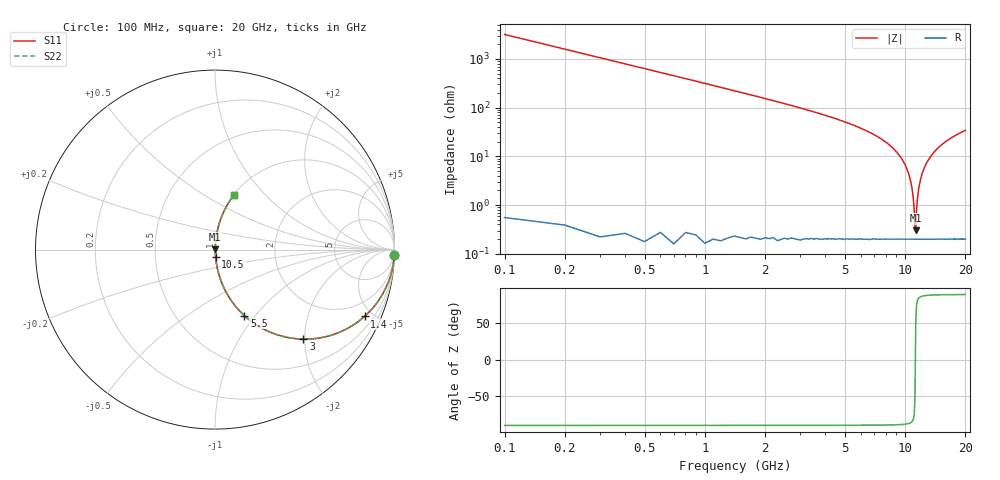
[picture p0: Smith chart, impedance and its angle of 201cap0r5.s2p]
! AVX Thin Film Operation		Date: May 2007
! Description: Accu-P® Series, Thin Film, SMD, RF Capacitor
! Part Number: 02013J0R5ABS
! 50 MHz  -  20.05 GHz
! Serial Measurements
# hz S db R 50
!	S11		S21		S12		S22
!	dB	Phase	dB	Phase	dB	Phase	dB	Phase
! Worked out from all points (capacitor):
!   200 points, 100 MHz to 20 GHz, reference 50 ohm
!   read as one part in series: C = 500 fF near 200 MHz
!   lowest |Z| = 305 mohm at 11.3 GHz (marker M1)
!   series resonance near 11.25 GHz, so ESL is about 400 pH
!   S11 on the Smith chart (normalised r, x): 100 MHz: 1, -64; 1.4 GHz: 1.00, -4.48; 3 GHz: 1.00, -1.97; 5.5 GHz: 1.00, -0.88; 10.5 GHz: 1.00, -0.08; 20 GHz: 1.00, +0.69
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1e8  -0.00 -1.8  -30.06 88.2  -30.06 88.2  -0.00 -1.8
3e8  -0.04 -5.4  -20.55 84.6  -20.55 84.6  -0.04 -5.4
5e8  -0.11 -8.9  -16.17 81.0  -16.17 81.0  -0.11 -8.9
1.4e9  -0.79 -24.1  -7.79 65.9  -7.79 65.9  -0.79 -24.1
3e9  -3.08 -45.4  -2.96 44.5  -2.96 44.5  -3.08 -45.4
3.5e9  -3.96 -50.5  -2.25 39.4  -2.25 39.4  -3.96 -50.5
5.5e9  -7.91 -66.0  -0.78 23.7  -0.78 23.7  -7.91 -66.0
6.8e9  -10.92 -73.1  -0.38 16.5  -0.38 16.5  -10.92 -73.1
8.8e9  -17.14 -81.2  -0.10 8.0  -0.10 8.0  -17.14 -81.2
1.01e10  -24.28 -84.6  -0.03 3.5  -0.03 3.5  -24.28 -84.6
1.05e10  -28.13 -84.8  -0.02 2.2  -0.02 2.2  -28.13 -84.8
1.09e10  -34.82 -82.7  -0.02 1.0  -0.02 1.0  -34.82 -82.7
1.11e10  -41.91 -75.2  -0.02 0.4  -0.02 0.4  -41.91 -75.2
1.12e10  -49.45 -53.5  -0.02 0.2  -0.02 0.2  -49.45 -53.5
1.13e10  -50.32 49.0  -0.02 -0.1  -0.02 -0.1  -50.32 49.0
1.14e10  -42.44 74.2  -0.02 -0.4  -0.02 -0.4  -42.44 74.2
1.15e10  -38.15 80.0  -0.02 -0.7  -0.02 -0.7  -38.15 80.0
1.18e10  -31.43 84.2  -0.02 -1.5  -0.02 -1.5  -31.43 84.2
1.24e10  -25.23 84.8  -0.03 -3.1  -0.03 -3.1  -25.23 84.8
1.34e10  -20.12 83.2  -0.06 -5.7  -0.06 -5.7  -20.12 83.2
1.67e10  -13.04 76.6  -0.24 -12.9  -0.24 -12.9  -13.04 76.6
2e10  -9.78 70.7  -0.50 -18.9  -0.50 -18.9  -9.78 70.7
